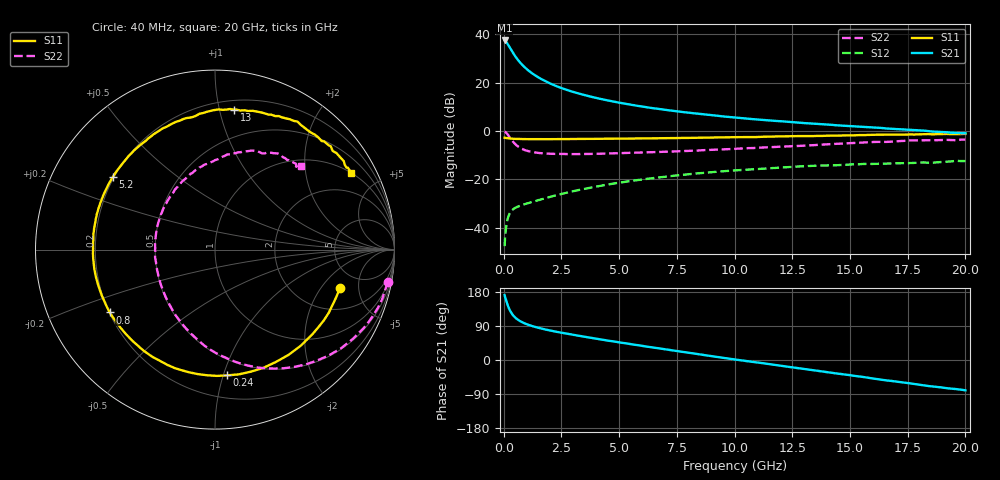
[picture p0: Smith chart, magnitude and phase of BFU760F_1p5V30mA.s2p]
! Filename:  P:\Prog\Test\Noise\ATS_data\Testdata_Net\Split files Spar\BFU760F_2W_C1_Bias7_1.5V_5mA_60mA_D.s2p
! Date/Time: Mon 06/Feb/2012 15:07:43
! BFU760_2W_C1_Bias7_1.5V_5mA_60mA_R.s2p
! MDIF S-parameter v. bias file
! BFU760_2W_C1_1.5V_5mA_60mA
! Date/time Fri Mar 18 11:09:37 2011
! VAR V_out= 1.5001
! VAR I_out= 29.9800
! VAR V_in= 0.7989
! VAR I_in= 0.0980
! Device data file deembeded for feedlines and parallel
! Original file: \Split files Spar\BFU760_2W_C1_Bias7_1.5V_5mA_60mA_R.s2p
! Feed-files: PR003V01_101208_Feed1.s2p, PR003V01_101208_Feed2.s2p
! Parallel-file: PR003V01_101208_Par.s2p
# MHz S MA R 50
!  Freq-MHz  S11-mag  S11-arg  S21-mag  S21-arg  S12-mag  S12-arg  S22-mag  S22-arg
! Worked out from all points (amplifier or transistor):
!   167 points, 40 MHz to 20 GHz, reference 50 ohm
!   highest |S21| = 37.5 dB at 40 MHz (marker M1)
!   |S21| within 3 dB of that: start of sweep to 269.1 MHz
!   unconditionally stable (mu >= 1): 3.732 GHz to 14.93 GHz
!   at 550 MHz: K = 0.34, MSG = 30.9 dB, |S12| = -31.6 dB
!   at 4.2 GHz: K = 1.02, MAG = 17.1 dB, |S12| = -22.6 dB
!   at 20 GHz: K = 0.93, MSG = 5.8 dB, |S12| = -12.4 dB
!   S11 on the Smith chart (normalised r, x): 40 MHz: 3.44, -3.10; 240 MHz: 0.37, -1.03; 800 MHz: 0.20, -0.27; 5.2 GHz: 0.20, +0.31; 13 GHz: 0.27, +1.11; 20 GHz: 0.99, +3.55
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40  0.7284 -16.9  74.86 171.1  0.004155 82.6  0.9795 -10.6
50  0.7258 -21.4  74.37 168.3  0.005224 85.3  0.9739 -13.8
90  0.72 -37.1  71.59 159.8  0.008973 74.2  0.9467 -25.1
140  0.7155 -55.0  66.81 150.2  0.01304 66.4  0.8913 -38.1
180  0.7118 -67.8  62.46 143.5  0.01576 61.0  0.8396 -47.4
240  0.7038 -84.5  56.02 134.7  0.01891 54.6  0.7647 -59.8
300  0.7003 -97.8  49.91 127.6  0.02126 49.8  0.697 -70.4
340  0.6973 -105.4  46.43 123.7  0.02243 47.4  0.6559 -76.6
460  0.6899 -123.0  37.65 114.3  0.02508 42.4  0.5618 -92.0
600  0.684 -136.4  30.34 106.9  0.02715 39.8  0.4878 -105.7
800  0.6829 -149.2  23.53 99.7  0.02955 38.6  0.4278 -120.5
1200  0.6802 -164.3  16.06 90.2  0.0339 39.8  0.3717 -140.4
1700  0.6804 -175.6  11.42 82.0  0.03971 42.1  0.3458 -156.2
2400  0.6812 174.0  8.073 73.2  0.04852 43.9  0.3361 -170.9
3400  0.6872 162.2  5.715 62.5  0.06246 43.5  0.3357 174.6
5200  0.6983 144.6  3.714 44.7  0.0884 37.8  0.3503 154.6
6800  0.7104 130.9  2.829 29.9  0.1109 30.1  0.3702 139.5
10200  0.7485 103.7  1.871 -0.1  0.1554 10.0  0.4345 111.1
13000  0.787 82.2  1.465 -23.6  0.1872 -8.1  0.4989 89.9
13400  0.7873 79.7  1.422 -26.8  0.191 -11.3  0.5105 87.0
16800  0.8427 54.0  1.111 -55.3  0.2135 -33.2  0.6041 62.6
20000  0.872 29.4  0.9024 -80.1  0.2396 -54.6  0.6672 44.2
